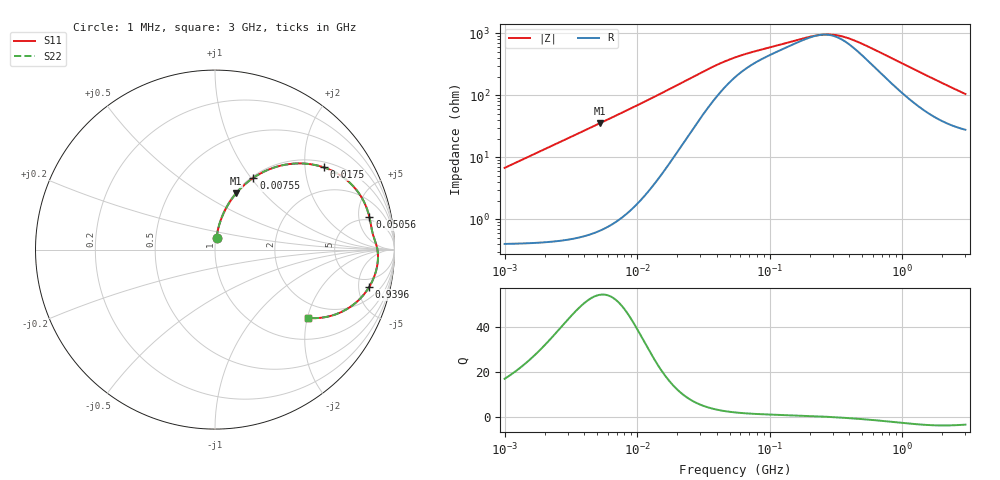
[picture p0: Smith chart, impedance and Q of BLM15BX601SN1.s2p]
! BLM15BX601SN1
# Hz S RI R 50
!Freq.(Hz) S11(Real) S11(Imag) S21(Real) S21(Imag) S12(Real) S12(Imag) S22(Real) S22(Imag)
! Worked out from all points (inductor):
!   401 points, 1 MHz to 3 GHz, reference 50 ohm
!   read as one part in series: L = 1.07 uH near 1.041 MHz
!   highest Q = 54.5 at 5.266 MHz (marker M1), where L = 1.08 uH
!   self-resonance near 245.7 MHz
!   S11 on the Smith chart (normalised r, x): 1 MHz: 1.01, +0.13; 7.55 MHz: 1.02, +1.03; 17.5 MHz: 1.16, +2.51; 50.56 MHz: 4.35, +6.92; 939.6 MHz: 3.46, -6.58; 3 GHz: 1.56, -2.03
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1000000  0.0084 0.0664  0.9916 -0.0664  0.9916 -0.0664  0.0084 0.0664
2014875  0.022 0.132  0.978 -0.132  0.978 -0.132  0.022 0.132
3823119  0.0666 0.2394  0.9334 -0.2394  0.9334 -0.2394  0.0666 0.2394
5266264  0.1172 0.3126  0.8828 -0.3126  0.8828 -0.3126  0.1172 0.3126
7550455  0.2143 0.4004  0.7857 -0.4004  0.7857 -0.4004  0.2143 0.4004
1.082539e7  0.3633 0.4671  0.6367 -0.4671  0.6367 -0.4671  0.3633 0.4671
1.461624e7  0.5155 0.4778  0.4845 -0.4778  0.4845 -0.4778  0.5155 0.4778
1.750132e7  0.6064 0.4581  0.3936 -0.4581  0.3936 -0.4581  0.6064 0.4581
2.270269e7  0.7186 0.3995  0.2814 -0.3995  0.2814 -0.3995  0.7186 0.3995
2.886629e7  0.7913 0.3283  0.2087 -0.3283  0.2087 -0.3283  0.7913 0.3283
3.74453e7  0.8368 0.2521  0.1632 -0.2521  0.1632 -0.2521  0.8368 0.2521
5.055795e7  0.8602 0.181  0.1398 -0.181  0.1398 -0.181  0.8602 0.181
5.477226e7  0.8636 0.1657  0.1364 -0.1657  0.1364 -0.1657  0.8636 0.1657
2.094008e8  0.9014 0.017  0.0986 -0.017  0.0986 -0.017  0.9014 0.017
2.771263e8  0.9068 -0.0136  0.0932 0.0136  0.0932 0.0136  0.9068 -0.0136
3.594878e8  0.9082 -0.0455  0.0918 0.0455  0.0918 0.0455  0.9082 -0.0455
4.75755e8  0.9046 -0.0848  0.0954 0.0848  0.0954 0.0848  0.9046 -0.0848
8.005644e8  0.8765 -0.1755  0.1235 0.1755  0.1235 0.1755  0.8765 -0.1755
9.395906e8  0.8588 -0.2084  0.1412 0.2084  0.1412 0.2084  0.8588 -0.2084
1.581072e9  0.7528 -0.32  0.2472 0.32  0.2472 0.32  0.7528 -0.32
2.221924e9  0.6377 -0.3713  0.3623 0.3713  0.3623 0.3713  0.6377 -0.3713
3e9  0.5197 -0.3809  0.4803 0.3809  0.4803 0.3809  0.5197 -0.3809
